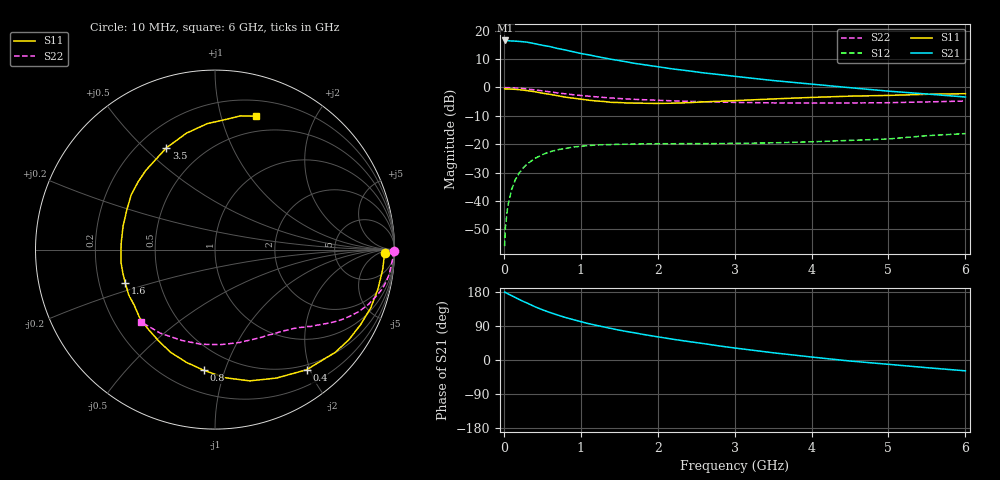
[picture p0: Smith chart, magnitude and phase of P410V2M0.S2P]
! SIEMENS Small Signal Semiconductors
! BFP182
! Si NPN RF Bipolar Junction Transistor in SOT143
! VCE = 10 V  IC = 2 mA
! Common Emitter S-Parameters:  March  1996
# GHz  S  MA  R  50
!  f  S11  S21  S12  S22
! GHz  MAG  ANG  MAG  ANG  MAG  ANG  MAG  ANG
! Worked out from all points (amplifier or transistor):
!   36 points, 10 MHz to 6 GHz, reference 50 ohm
!   highest |S21| = 16.6 dB at 20 MHz (marker M1)
!   |S21| within 3 dB of that: start of sweep to 732.2 MHz
!   unconditionally stable (mu >= 1): 2.25 GHz to end of sweep
!   at 250 MHz: K = 0.12, MSG = 22.3 dB, |S12| = -28.4 dB
!   at 1.4 GHz: K = 0.66, MSG = 15.0 dB, |S12| = -20.1 dB
!   at 6 GHz: K = 1.02, MAG = 5.6 dB, |S12| = -16.3 dB
!   S11 on the Smith chart (normalised r, x): 10 MHz: 31, -13; 400 MHz: 0.42, -1.95; 800 MHz: 0.34, -0.85; 1.6 GHz: 0.31, -0.16; 3.5 GHz: 0.31, +0.58; 6 GHz: 0.34, +1.29
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0.01  0.9467 -1.3  6.687 179.0  0.0016 79.6  0.9951 -0.5
0.02  0.9429 -2.8  6.733 178.4  0.0034 87.3  0.9916 -1.0
0.05  0.9409 -6.8  6.681 174.9  0.008 87.7  0.9923 -2.7
0.1  0.9338 -13.7  6.587 169.9  0.0157 80.7  0.9855 -5.4
0.15  0.9265 -20.5  6.548 164.8  0.0238 77.5  0.9802 -8.1
0.25  0.899 -34.0  6.384 154.8  0.038 70.2  0.9571 -13.2
0.3  0.8812 -40.5  6.291 150.5  0.0445 66.1  0.9397 -15.5
0.4  0.8416 -52.7  5.916 141.0  0.0559 59.9  0.9075 -19.7
0.5  0.7936 -64.4  5.543 132.7  0.0655 53.4  0.8716 -23.4
0.6  0.7566 -75.2  5.256 125.3  0.0737 48.1  0.8356 -26.5
0.8  0.6753 -95.3  4.574 112.2  0.0843 39.2  0.7715 -31.6
1  0.6232 -113.5  3.971 101.2  0.0921 32.9  0.7222 -35.3
1.1  0.5971 -122.0  3.764 96.0  0.0947 30.2  0.7016 -37.0
1.3  0.5664 -137.7  3.32 87.2  0.0979 25.4  0.6671 -40.0
1.6  0.5334 -159.5  2.815 75.1  0.1005 20.6  0.6284 -44.1
1.9  0.5244 -177.9  2.43 64.6  0.1016 17.4  0.6024 -48.2
2.2  0.5285 165.7  2.117 54.7  0.102 15.5  0.5813 -52.4
2.8  0.5712 138.5  1.687 37.1  0.103 13.5  0.5531 -62.0
3.5  0.628 115.6  1.326 19.1  0.1058 13.9  0.5352 -75.3
4.5  0.7033 93.5  0.991 -2.7  0.1168 15.4  0.5332 -98.3
5.5  0.7585 79.2  0.767 -20.3  0.1414 16.6  0.5566 -123.3
6  0.7771 73.0  0.679 -28.6  0.1539 14.0  0.5766 -135.7
